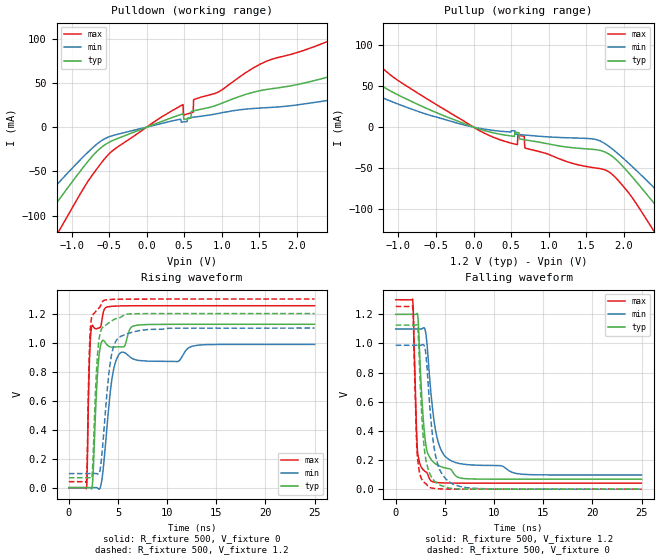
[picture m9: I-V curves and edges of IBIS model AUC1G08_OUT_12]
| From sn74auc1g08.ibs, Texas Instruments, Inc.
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[Model]   AUC1G08_OUT_12
Model_type  Output
Vref =   0
Rref =   2000
Cref =   15p
Vmeas =   0.6
| variable   typ   min   max
C_comp   6.75pF   1.50pF   15.58pF
| C_pullup   5.97pF   1.50pF   11.79pF
| C_pulldown   7.54pF   4.82pF   15.58pF
[Temperature Range]   40   100   -40
| Ambient temperature   25   85   -40
[Voltage range]   1.2   1.1   1.3
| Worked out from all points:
|   slope of the pulldown table from 0 to 0.18 V, typ, clamps not added: 31 ohm
|   slope of the pullup table from 0 to 0.18 V, typ, clamps not added: 35.6 ohm
|   rising waveform, R_fixture 500, V_fixture 0: 20-80 % time 511ps typ, 891ps min, 276ps max; typ from 0 V to 1.13 V
|   falling waveform, R_fixture 500, V_fixture 1.2: 20-80 % time 681ps typ, 1.15ns min, 334ps max; typ from 1.2 V to 0.068 V
|   rising waveform, R_fixture 500, V_fixture 1.2: 20-80 % time 480ps typ, 849ps min, 259ps max; typ from 0.068 V to 1.2 V
|   falling waveform, R_fixture 500, V_fixture 0: 20-80 % time 619ps typ, 929ps min, 329ps max; typ from 1.13 V to 0 V
[Pulldown]
| AUC1G08_OUT_12
|   Voltage   I(typ)   I(min)   I(max)
-3.6V     -362.2mA   -295.5mA   -456.7mA
-1.955V   -173.1mA   -136.4mA   -229.6mA
-1.425V   -111.8mA   -86.22mA   -154.8mA
-1.27V    -93.84mA   -71.79mA   -132.4mA
-460mV    -15.42mA   -9.769mA   -27.03mA
485mV     15.08mA    5.877mA    25.53mA
620mV     18.29mA    11.19mA    16.89mA
630mV     18.49mA    11.3mA     31.2mA
1.525V    41.46mA    21.67mA    71.78mA
2.85V     66.35mA    26.32mA    111.9mA
3.56V     55.29mA    27.59mA    134.2mA
7.2V      68.67mA    34.86mA    121.5mA
[Pullup]
| AUC1G08_OUT_12
|   Voltage   I(typ)   I(min)   I(max)
-3.6V     232.3mA    103.4mA    299.9mA
-2.99V    183.5mA    84.99mA    240.2mA
-2.35V    130.5mA    94.06mA    177.7mA
-1.85V    91.83mA    66.12mA    129.7mA
-1.045V   41.24mA    29.65mA    59.59mA
130mV     -3.803mA   -2.249mA   -6.7mA
675mV     -15.4mA    -9.612mA   -11.23mA
1.785V    -31.98mA   -22.32mA   -53.69mA
2.39V     -91.47mA   -72.72mA   -125.4mA
2.665V    -122.9mA   -98.03mA   -165.3mA
2.975V    -158.7mA   -127.3mA   -210mA
7.2V      -650.8mA   -541mA     -806.2mA
[Ramp]
| AUC1G08_OUT_12
| variable   typ   min   max
dV/dt_r   0.68/5.17E-10   0.60/8.98E-10   0.76/2.78E-10
dV/dt_f   0.68/6.86E-10   0.61/1.15E-09   0.76/3.38E-10
R_load = 500
[Rising Waveform]
| AUC1G08_OUT_12
R_fixture =   500
C_fixture =   0
L_fixture =   0
V_fixture =   0
V_fixture_min = 0
V_fixture_max = 0
|   Time   V(typ)   V(min)   V(max)
0s        5.277nV    22.79nV    363.9pV
1.795ns   -5.224uV   -3.174uV   -3.647mV
2.105ns   655.7uV    -8.955uV   883.7mV
2.365ns   848.2uV    -10.71uV   1.118V
3.025ns   877.6mV    -8.444mV   1.1V
3.73ns    998.3mV    297mV      1.24V
4.45ns    968.6mV    776mV      1.25V
5.32ns    970.8mV    932.1mV    1.253V
7.03ns    1.121V     877.3mV    1.254V
24.99ns   1.126V     987.6mV    1.254V
[Falling Waveform]
| AUC1G08_OUT_12
R_fixture =   500
C_fixture =   0
L_fixture =   0
V_fixture =   1.2
V_fixture_min = 1.1
V_fixture_max = 1.3
|   Time   V(typ)   V(min)   V(max)
0s        1.2V       1.1V       1.3V
1.725ns   1.2V       1.1V       1.304V
1.795ns   1.2V       1.1V       1.218V
2.21ns    1.206V     1.1V       266.9mV
2.905ns   399.7mV    1.107V     126.6mV
3.14ns    275.6mV    1.027V     115.3mV
3.615ns   203.2mV    638.8mV    55.9mV
4.43ns    159.4mV    300.4mV    44.5mV
5.925ns   105.1mV    186.6mV    41.69mV
24.99ns   68.46mV    97.32mV    41.2mV
[Rising Waveform]
| AUC1G08_OUT_12
R_fixture =   500
C_fixture =   0
L_fixture =   0
V_fixture =   1.2
V_fixture_min = 1.1
V_fixture_max = 1.3
|   Time   V(typ)   V(min)   V(max)
0s        68.42mV    97.28mV    41.19mV
1.785ns   68.42mV    97.28mV    34.79mV
1.85ns    68.42mV    97.28mV    125.7mV
2.085ns   68.84mV    97.28mV    926.7mV
2.32ns    66.43mV    97.27mV    1.174V
2.93ns    925.1mV    94.28mV    1.23V
3.515ns   1.11V      346.8mV    1.288V
4.295ns   1.147V     896.2mV    1.297V
5.3ns     1.175V     1.043V     1.299V
24.99ns   1.2V       1.1V       1.3V
[Falling Waveform]
| AUC1G08_OUT_12
R_fixture =   500
C_fixture =   0
L_fixture =   0
V_fixture =   0
V_fixture_min = 0
V_fixture_max = 0
|   Time   V(typ)   V(min)   V(max)
0s        1.126V     987.6mV    1.254V
1.725ns   1.126V     987.6mV    1.256V
2.09ns    1.128V     987.6mV    395.2mV
2.21ns    1.127V     987.5mV    222.3mV
2.79ns    366.5mV    992.1mV    54.66mV
3.06ns    205.3mV    931.9mV    37.92mV
3.365ns   125.3mV    660.5mV    15.95mV
4.185ns   41.16mV    191.9mV    3.499mV
5.86ns    3.382mV    33.85mV    418uV
24.99ns   33.67uV    10.48uV    13.81uV
